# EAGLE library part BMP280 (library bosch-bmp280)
The BMP280 is an absolute barometric pressure sensor especially designed for mobile applications. The sensor module is housed in an extremely compact 8-pin metal-lid LGA package with a footprint of only 2.0 × 2.5 mm2 and 0.95 mm package height. Its small dimensions and its low power consumption of 2.7 μA @1Hz allow the implementation in battery driven devices such as mobile phones, GPS modules or watches. The library has been designed by Richard Magdycz
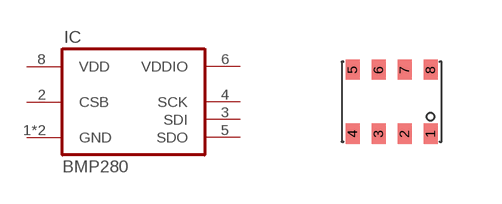
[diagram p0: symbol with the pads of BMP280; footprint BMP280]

Designator prefix IC

## BMP280  [BMP280]
1  GND  pwr
2  CSB  in
3  SDI
4  SCK
5  SDO  in
6  VDDIO  pwr
7  GND  pwr
8  VDD  pwr

## Footprint BMP280 (pad centres in mm)
2.5 mm x 2.5 mm x 0.93 mm metal lid LGA
smd 0.35 x 0.5: 1 0.975,-0.8; 2 0.325,-0.8; 3 -0.325,-0.8; 4 -0.975,-0.8; 5 -0.975,0.8; 6 -0.325,0.8; 7 0.325,0.8; 8 0.975,0.8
